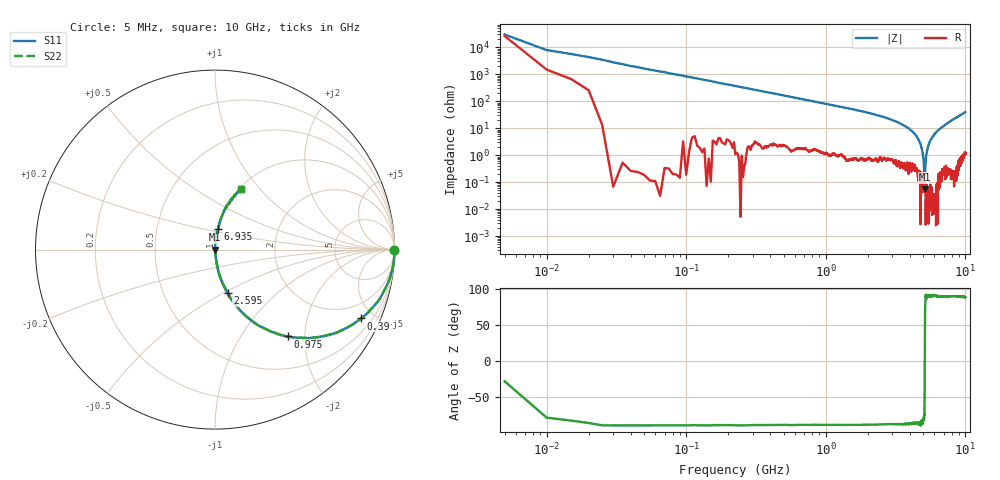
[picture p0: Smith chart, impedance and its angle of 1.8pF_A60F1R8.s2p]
! Amotech Co.,Ltd.
! http://www.amotech.co.kr/
! Part Number: A60F1R8
! These Parameters are Measured in Series Mode Connection
! Operation Temp=25[degC], DC Bias Voltage=0[V]
! Freq. Start=5[MHz] Stop=10[GHz], 2000[Steps]
! Date: Monday, July 20, 2020, 03:17:25
# GHZ S RI R 50.000000
!Freq.(Hz) S11(Real) S11(Imag) S21(Real) S21(Imag) S12(Real) S12(Imag) S22(Real) S22(Imag)
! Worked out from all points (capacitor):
!   2000 points, 5 MHz to 10 GHz, reference 50 ohm
!   read as one part in series: C = 1.91 pF near 55 MHz
!   lowest |Z| = 55.4 mohm at 5.12 GHz (marker M1)
!   series resonance near 5.114 GHz, so ESL is about 510 pH
!   S11 on the Smith chart (normalised r, x): 5 MHz: open; 390 MHz: 1.04, -4.23; 975 MHz: 1.02, -1.65; 2.595 GHz: 1.02, -0.52; 6.935 GHz: 1.00, +0.24; 10 GHz: 1.02, +0.80
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0.005  0.9971 -0.00159  0.00292 0.00159  0.00292 0.00159  0.9971 -0.00159
0.06  0.9948 -0.0719  0.00521 0.0719  0.00521 0.0719  0.9948 -0.0719
0.11  0.9824 -0.1285  0.0176 0.1285  0.0176 0.1285  0.9824 -0.1285
0.22  0.933 -0.246  0.067 0.246  0.067 0.246  0.933 -0.246
0.39  0.8148 -0.3833  0.1852 0.3833  0.1852 0.3833  0.8148 -0.3833
0.975  0.4068 -0.4841  0.5932 0.4841  0.5932 0.4841  0.4068 -0.4841
1.675  0.1826 -0.3791  0.8174 0.3791  0.8174 0.3791  0.1826 -0.3791
2.595  0.0703 -0.2415  0.9297 0.2415  0.9297 0.2415  0.0703 -0.2415
3.34  0.03 -0.1525  0.97 0.1525  0.97 0.1525  0.03 -0.1525
4.485  0.00536 -0.0488  0.9946 0.0488  0.9946 0.0488  0.00536 -0.0488
4.8  0.00162 -0.0231  0.9984 0.0231  0.9984 0.0231  0.00162 -0.0231
4.93  0.000801 -0.0132  0.9992 0.0132  0.9992 0.0132  0.000801 -0.0132
5.005  0.00138 -0.00725  0.9986 0.00725  0.9986 0.00725  0.00138 -0.00725
5.08  0.000537 -0.00202  0.9995 0.00202  0.9995 0.00202  0.000537 -0.00202
5.12  0.000533 0.000148  0.9995 -0.000148  0.9995 -0.000148  0.000533 0.000148
5.23  -4.84e-05 0.00934  1 -0.00934  1 -0.00934  -4.84e-05 0.00934
5.425  0.000489 0.0229  0.9995 -0.0229  0.9995 -0.0229  0.000489 0.0229
5.835  0.00211 0.0504  0.9979 -0.0504  0.9979 -0.0504  0.00211 0.0504
6.67  0.0126 0.1012  0.9874 -0.1012  0.9874 -0.1012  0.0126 0.1012
6.935  0.0162 0.1175  0.9838 -0.1175  0.9838 -0.1175  0.0162 0.1175
8.335  0.0515 0.2178  0.9485 -0.2178  0.9485 -0.2178  0.0515 0.2178
10  0.145 0.3371  0.855 -0.3371  0.855 -0.3371  0.145 0.3371
